| TEXAS INSTRUMENTS INCORPORATED
| Standard Linear and Logic Group
| IBIS Model of SN74AHC14
| HEX SCHMITT-TRIGGER INVERTERS
| This file contains package information for the following:
|  SOIC 14-pin (D) package as [Component] AHC14_D
|  PDIP 14-pin (N) package as [Component] AHC14_N
|  SOP 14-pin (NS) package as [Component] AHC14_NS
|  SSOP 14-pin (DB) package as [Component] AHC14_DB
|  TSSOP 14-pin (PW) package as [Component] AHC14_PW
|  TVSOP 14-pin (DGV) package as [Component] AHC14_DGV
| This device can be powered at the following Vccs:
|  2.2 volt Vcc
|  3.3 volt Vcc
|  5 volt Vcc
| This file provides unique models under the [Model Selector] for each Vcc.
| For operation at a specific Vcc, select the appropriate model after each
| [Model Selector] keyword.
[IBIS Ver]   3.2
[Comment char]  |_char
[File Name]   sn74ahc14.ibs
[File Rev]   1.1 | b_die
[Date]   June 7, 2002
[Source]   Data created from TI-SPICE simulations at TI-SLL.
[Notes]   The following is an IBIS list for the SN74AHC14.
   Please contact sllibis@ti.com with questions and
   comments concerning SLL IBIS models.
   This IBIS model is created from a BA (back annotated netlist).
[Disclaimer] Property of Texas Instruments Incorporated.  Unauthorized
   reproduction and/or distribution is strictly prohibited.
   This product is protected under copyright law.
   Created 2002, (C) Copyright 2002, Texas Instruments
   Incorporated, All Rights Reserved
   UNLESS THERE IS A SIGNED, WRITTEN AGREEMENT TO THE
   CONTRARY, TEXAS INSTRUMENTS (TI) IS PROVIDING THE IBIS
   MODELS AND WITHOUT ANY WARRANTY, EXPRESSED OR
   IMPLIED. TI assumes no liability for:
   1) the accuracy of the IBIS models provided to your
   company;
   2) the proper functioning of these IBIS Models in your
   design or for any resulting applications; or
   3) infringement of patents, copyrights or intellectual
   property rights resulting from your use of these IBIS
   models.
   TI provides IBIS Models as a service to our customers.
   You and your company shall not distribute, sell or give
   these models to anyone else without prior written
   permission from TI.
   TI reserves the right to make changes to our products or
   to discontinue any semiconductor product or service
   without notice, and advises our customers to obtain the
   latest version of relevant information to verify, before
   placing orders, that the information being relied on is
   current.
   Please be aware that your receipt and use of the IBIS
   information provided shall serve as acceptance of these
   terms and conditions. If you do not accept these terms,
   you should return or destroy the IBIS models and any
   other accompanying information immediately.
| Component AHC14_D 14-pin SOIC
[Component]   AHC14_D
[Manufacturer]   Texas Instruments, Inc.
[Package]
|   typ   min   max
R_pkg   3.100e-02   2.800e-02   3.400e-02
L_pkg   3.109e-09   2.462e-09   3.889e-09
C_pkg   4.730e-13   3.630e-13   6.280e-13
[Pin]   signal_name   model_name   R_pin   L_pin   C_pin
1   1A   AHC14_IN   3.300e-02   3.854e-09   6.220e-13
2   1Y   AHC14_OUT   3.200e-02   3.188e-09   4.730e-13
3   2A   AHC14_IN   2.800e-02   2.462e-09   3.770e-13
4   2Y   AHC14_OUT   3.100e-02   2.596e-09   3.630e-13
5   3A   AHC14_IN   2.800e-02   2.521e-09   3.720e-13
6   3Y   AHC14_OUT   3.400e-02   3.250e-09   4.760e-13
7   GND   GND   3.400e-02   3.889e-09   6.280e-13
8   4Y   AHC14_OUT   3.400e-02   3.889e-09   6.280e-13
9   4A   AHC14_IN   3.400e-02   3.250e-09   4.760e-13
10   5Y   AHC14_OUT   2.800e-02   2.521e-09   3.720e-13
11   5A   AHC14_IN   3.100e-02   2.596e-09   3.640e-13
12   6Y   AHC14_OUT   2.800e-02   2.462e-09   3.770e-13
13   6A   AHC14_IN   3.200e-02   3.188e-09   4.730e-13
14   VCC   POWER   3.300e-02   3.854e-09   6.220e-13
| Component AHC14_N 14-pin PDIP
[Component]   AHC14_N
[Manufacturer]   Texas Instruments, Inc.
[Package]
|   typ   min   max
R_pkg   4.500e-02   3.700e-02   6.300e-02
L_pkg   5.407e-09   3.922e-09   6.942e-09
C_pkg   3.890e-13   2.050e-13   6.040e-13
[Pin]   signal_name   model_name   R_pin   L_pin   C_pin
1   1A   AHC14_IN   6.300e-02   6.942e-09   6.040e-13
2   1Y   AHC14_OUT   3.700e-02   6.200e-09   4.060e-13
3   2A   AHC14_IN   4.200e-02   4.389e-09   3.220e-13
4   2Y   AHC14_OUT   3.800e-02   3.922e-09   2.050e-13
5   3A   AHC14_IN   3.900e-02   4.301e-09   2.980e-13
6   3Y   AHC14_OUT   3.800e-02   5.329e-09   3.560e-13
7   GND   GND   5.300e-02   6.510e-09   5.440e-13
8   4Y   AHC14_OUT   5.300e-02   6.437e-09   5.390e-13
9   4A   AHC14_IN   3.900e-02   5.352e-09   3.470e-13
10   5Y   AHC14_OUT   4.200e-02   4.473e-09   2.970e-13
11   5A   AHC14_IN   4.400e-02   4.326e-09   2.250e-13
12   6Y   AHC14_OUT   4.200e-02   4.295e-09   2.800e-13
13   6A   AHC14_IN   4.200e-02   6.318e-09   4.180e-13
14   VCC   POWER   6.100e-02   6.900e-09   6.030e-13
| Component AHC14_NS 14-pin SOP
[Component]   AHC14_NS
[Manufacturer]   Texas Instruments, Inc.
[Package]
|   typ   min   max
R_pkg   4.500e-02   3.900e-02   5.400e-02
L_pkg   3.796e-09   2.561e-09   4.952e-09
C_pkg   5.280e-13   2.880e-13   7.100e-13
[Pin]   signal_name   model_name   R_pin   L_pin   C_pin
1   1A   AHC14_IN   4.700e-02   4.867e-09   7.060e-13
2   1Y   AHC14_OUT   5.100e-02   4.083e-09   5.920e-13
3   2A   AHC14_IN   4.100e-02   2.915e-09   3.760e-13
4   2Y   AHC14_OUT   3.900e-02   2.561e-09   2.880e-13
5   3A   AHC14_IN   4.100e-02   3.101e-09   4.300e-13
6   3Y   AHC14_OUT   4.700e-02   4.047e-09   5.890e-13
7   GND   GND   5.100e-02   4.909e-09   7.000e-13
8   4Y   AHC14_OUT   4.500e-02   4.784e-09   6.940e-13
9   4A   AHC14_IN   5.400e-02   4.176e-09   5.970e-13
10   5Y   AHC14_OUT   3.900e-02   3.287e-09   4.490e-13
11   5A   AHC14_IN   3.900e-02   2.586e-09   2.940e-13
12   6Y   AHC14_OUT   4.000e-02   2.802e-09   3.710e-13
13   6A   AHC14_IN   4.900e-02   4.080e-09   5.930e-13
14   VCC   POWER   5.200e-02   4.952e-09   7.100e-13
| Component AHC14_DB 14-pin SSOP
[Component]   AHC14_DB
[Manufacturer]   Texas Instruments, Inc.
[Package]
|   typ   min   max
R_pkg   4.400e-02   4.100e-02   4.600e-02
L_pkg   3.551e-09   3.258e-09   3.927e-09
C_pkg   4.020e-13   3.600e-13   4.210e-13
[Pin]   signal_name   model_name   R_pin   L_pin   C_pin
1   1A   AHC14_IN   4.600e-02   3.927e-09   4.080e-13
2   1Y   AHC14_OUT   4.400e-02   3.587e-09   4.210e-13
3   2A   AHC14_IN   4.100e-02   3.289e-09   3.980e-13
4   2Y   AHC14_OUT   4.200e-02   3.258e-09   3.600e-13
5   3A   AHC14_IN   4.100e-02   3.286e-09   4.030e-13
6   3Y   AHC14_OUT   4.400e-02   3.586e-09   4.210e-13
7   GND   GND   4.600e-02   3.927e-09   4.080e-13
8   4Y   AHC14_OUT   4.600e-02   3.927e-09   4.080e-13
9   4A   AHC14_IN   4.400e-02   3.586e-09   4.210e-13
10   5Y   AHC14_OUT   4.100e-02   3.286e-09   4.030e-13
11   5A   AHC14_IN   4.300e-02   3.258e-09   3.600e-13
12   6Y   AHC14_OUT   4.100e-02   3.289e-09   3.980e-13
13   6A   AHC14_IN   4.400e-02   3.587e-09   4.210e-13
14   VCC   POWER   4.600e-02   3.927e-09   4.080e-13
| Component AHC14_PW 14-pin TSSOP
[Component]   AHC14_PW
[Manufacturer]   Texas Instruments, Inc.
[Package]
|   typ   min   max
R_pkg   3.200e-02   2.900e-02   3.500e-02
L_pkg   2.378e-09   2.170e-09   2.680e-09
C_pkg   3.140e-13   2.700e-13   3.350e-13
[Pin]   signal_name   model_name   R_pin   L_pin   C_pin
1   1A   AHC14_IN   3.300e-02   2.618e-09   3.300e-13
2   1Y   AHC14_OUT   3.100e-02   2.313e-09   3.170e-13
3   2A   AHC14_IN   3.000e-02   2.310e-09   3.140e-13
4   2Y   AHC14_OUT   3.100e-02   2.173e-09   2.720e-13
5   3A   AHC14_IN   3.000e-02   2.204e-09   3.090e-13
6   3Y   AHC14_OUT   3.200e-02   2.315e-09   3.170e-13
7   GND   GND   3.500e-02   2.680e-09   3.350e-13
8   4Y   AHC14_OUT   3.300e-02   2.640e-09   3.330e-13
9   4A   AHC14_IN   3.400e-02   2.347e-09   3.190e-13
10   5Y   AHC14_OUT   2.900e-02   2.277e-09   3.130e-13
11   5A   AHC14_IN   3.100e-02   2.170e-09   2.700e-13
12   6Y   AHC14_OUT   3.100e-02   2.244e-09   3.110e-13
13   6A   AHC14_IN   3.300e-02   2.343e-09   3.210e-13
14   VCC   POWER   3.500e-02   2.657e-09   3.320e-13
| Component AHC14_DGV 14-pin TVSOP
[Component]   AHC14_DGV
[Manufacturer]   Texas Instruments, Inc.
[Package]
|   typ   min   max
R_pkg   3.500e-02   2.000e-02   4.500e-02
L_pkg   2.499e-09   2.077e-09   2.966e-09
C_pkg   3.610e-13   3.050e-13   4.160e-13
[Pin]   signal_name   model_name   R_pin   L_pin   C_pin
1   1A   AHC14_IN   2.700e-02   2.717e-09   3.730e-13
2   1Y   AHC14_OUT   3.700e-02   2.434e-09   3.980e-13
3   2A   AHC14_IN   3.400e-02   2.200e-09   3.160e-13
4   2Y   AHC14_OUT   2.000e-02   2.077e-09   3.090e-13
5   3A   AHC14_IN   3.000e-02   2.147e-09   3.050e-13
6   3Y   AHC14_OUT   4.200e-02   2.580e-09   4.080e-13
7   GND   GND   3.900e-02   2.921e-09   3.850e-13
8   4Y   AHC14_OUT   3.300e-02   2.841e-09   3.800e-13
9   4A   AHC14_IN   4.200e-02   2.611e-09   4.100e-13
10   5Y   AHC14_OUT   3.800e-02   2.331e-09   3.290e-13
11   5A   AHC14_IN   2.600e-02   2.223e-09   3.190e-13
12   6Y   AHC14_OUT   3.400e-02   2.259e-09   3.130e-13
13   6A   AHC14_IN   4.500e-02   2.681e-09   4.160e-13
14   VCC   POWER   4.200e-02   2.966e-09   3.860e-13
| Model AHC14_IN
[Model Selector]   AHC14_IN
AHC14_IN_22   2.2 volt Vcc
AHC14_IN_33   3.3 volt Vcc
AHC14_IN_50   5 volt Vcc
| Model AHC14_OUT
[Model Selector]   AHC14_OUT
AHC14_OUT_22   2.2 volt Vcc
AHC14_OUT_33   3.3 volt Vcc
AHC14_OUT_50   5 volt Vcc
| Models and submodels in the file (6): AHC14_IN_22 (Input), AHC14_IN_33 (Input), AHC14_IN_50 (Input), AHC14_OUT_22 (Output), AHC14_OUT_33 (Output), AHC14_OUT_50 (Output)
